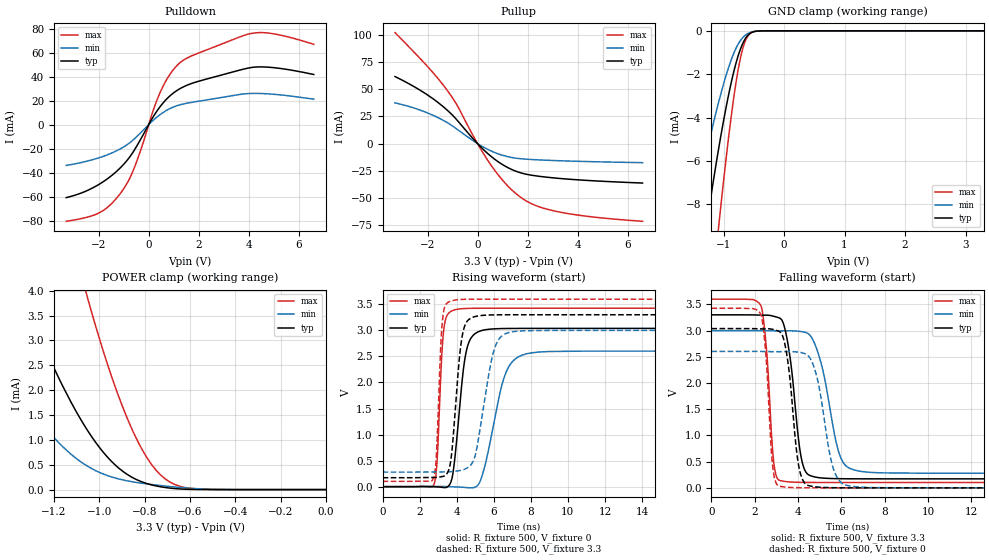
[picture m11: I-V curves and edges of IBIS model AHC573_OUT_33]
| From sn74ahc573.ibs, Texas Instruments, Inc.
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[Model]   AHC573_OUT_33
Model_type  3-state
Enable   Active-Low
Vref =   0.0
Rref =   1000
Cref =   50p
Vmeas =   1.65
| variable   typ   min   max
C_comp   2.19pF   1.91pF   2.36pF
| C_pullup   3.29pF   2.02pF   4.04pF
| C_pulldown   2.75pF   1.99pF   3.57pF
| C_tri-state   2.19pF   1.91pF   2.36pF
[Temperature Range]   40   100   -40
| Ambient temperature   25   85   -40
[Voltage range]   3.3   3   3.6
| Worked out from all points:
|   slope of the pulldown table from 0 to 0.495 V, typ, clamps not added: 30.9 ohm
|   slope of the pullup table from 0 to 0.495 V, typ, clamps not added: 45.5 ohm
|   GND clamp passes 1 mA (typ) near -0.74 V on its own axis
|   POWER clamp passes 1 mA (typ) near -1.02 V on its own axis
|   rising waveform, R_fixture 500, V_fixture 0: 20-80 % time 514ps typ, 946ps min, 263ps max; typ from 0 V to 3.04 V
|   falling waveform, R_fixture 500, V_fixture 3.3: 20-80 % time 499ps typ, 776ps min, 325ps max; typ from 3.3 V to 0.172 V
|   rising waveform, R_fixture 500, V_fixture 3.3: 20-80 % time 436ps typ, 764ps min, 239ps max; typ from 0.172 V to 3.3 V
|   falling waveform, R_fixture 500, V_fixture 0: 20-80 % time 439ps typ, 642ps min, 297ps max; typ from 3.04 V to 0 V
[GND Clamp]
| AHC573_OUT_33
|   Voltage   I(typ)   I(min)   I(max)
-3.3V     -60.86mA   -39.73mA   -82.26mA
-1.52V    -13.86mA   -8.821mA   -21.9mA
-1.28V    -8.984mA   -5.626mA   -14.64mA
-1.1V     -5.753mA   -3.504mA   -9.558mA
-1.07V    -5.258mA   -3.179mA   -8.754mA
-905mV    -2.803mA   -1.596mA   -4.662mA
-835mV    -1.937mA   -1.066mA   -3.167mA
-780mV    -1.355mA   -728.6uA   -2.148mA
-690mV    -630uA     -338.2uA   -897.4uA
-590mV    -183.7uA   -113uA     -211.6uA
-375mV    -3.862uA   -2.975uA   -1.96uA
3.3V      10.72nA    15.77nA    51.49nA
[POWER Clamp]
| AHC573_OUT_33
|   Voltage   I(typ)   I(min)   I(max)
-3.3V     44.46mA    27.37mA    76.31mA
-1.605V   7.526mA    3.914mA    16.22mA
-1.335V   3.908mA    1.826mA    9.462mA
-1.18V    2.261mA    949.9uA    6.178mA
-1.065V   1.287mA    509.3uA    4.083mA
-1.05V    1.179mA    466.7uA    3.834mA
-960mV    635.2uA    276.2uA    2.471mA
-865mV    272.4uA    166.5uA    1.311mA
-790mV    121.4uA    114.1uA    643.8uA
-710mV    42.77uA    72.33uA    217.8uA
-575mV    2.489uA    19.9uA     14.31uA
-48.03fV  10.72nA    1.614nA    79.93nA
[Pulldown]
| AHC573_OUT_33
|   Voltage   I(typ)   I(min)   I(max)
-3.3V     -60.82mA   -34mA      -80.56mA
-1.955V   -49.36mA   -27.41mA   -73.22mA
-1.53V    -43.23mA   -24.12mA   -66.71mA
-1.095V   -35.12mA   -19.74mA   -56.23mA
-580mV    -21.4mA    -11.96mA   -36.16mA
195mV     7.045mA    3.905mA    12.83mA
505mV     16.27mA    9.059mA    28.99mA
905mV     24.95mA    13.91mA    43.54mA
1.345V    31mA       17.03mA    53.09mA
4.23V     47.88mA    26mA       76.33mA
5.125V    47.14mA    25.02mA    75.15mA
6.6V      41.74mA    21.26mA    66.86mA
[Pullup]
| AHC573_OUT_33
|   Voltage   I(typ)   I(min)   I(max)
-3.3V     61.59mA    37.44mA    102mA
-2.18V    47.37mA    29.8mA     75.34mA
-1.31V    32.68mA    20.57mA    51.94mA
-830mV    21.86mA    13.38mA    35.7mA
-40mV     989.5uA    591.7uA    1.624mA
495mV     -10.88mA   -6.291mA   -18.35mA
1.08V     -20.42mA   -11.28mA   -35.71mA
1.66V     -26.4mA    -13.78mA   -48.23mA
2.305V    -29.58mA   -14.83mA   -56.72mA
3.225V    -31.92mA   -15.73mA   -62.67mA
4.61V     -34.17mA   -16.65mA   -67.45mA
6.6V      -36.27mA   -17.55mA   -71.43mA
[Ramp]
| AHC573_OUT_33
| variable   typ   min   max
dV/dt_r   1.83/5.21E-10   1.58/9.54E-10   2.06/2.67E-10
dV/dt_f   1.88/5.01E-10   1.63/7.78E-10   2.10/3.30E-10
R_load = 500
[Rising Waveform]
| AHC573_OUT_33
R_fixture =   500
C_fixture =   0
L_fixture =   0
V_fixture =   0
V_fixture_min = 0
V_fixture_max = 0
|   Time   V(typ)   V(min)   V(max)
0s        717.3pV    1.212nV    402.8pV
2.775ns   -836.6uV   4.547mV    44.17mV
2.94ns    -4.688mV   4.776mV    497mV
3.315ns   -17.22mV   3.17mV     3.053V
4ns       903mV      -5.604mV   3.404V
4.405ns   2.371V     -14.01mV   3.419V
4.785ns   2.861V     -22.99mV   3.423V
6.695ns   3.036V     2.223V     3.425V
8.005ns   3.038V     2.567V     3.425V
50ns      3.038V     2.603V     3.425V
[Falling Waveform]
| AHC573_OUT_33
R_fixture =   500
C_fixture =   0
L_fixture =   0
V_fixture =   3.3
V_fixture_min = 3
V_fixture_max = 3.6
|   Time   V(typ)   V(min)   V(max)
0s        3.3V       3V         3.6V
2.305ns   3.294V     3V         3.456V
2.875ns   3.273V     2.995V     491.4mV
3.21ns    3.22V      2.995V     134mV
3.605ns   2.558V     2.996V     113.2mV
4.185ns   498.8mV    2.979V     105mV
4.905ns   198mV      2.595V     102.7mV
5.94ns    174.7mV    605.7mV    102.1mV
7.005ns   172.1mV    307.7mV    102mV
50ns      171.7mV    279.8mV    102mV
[Rising Waveform]
| AHC573_OUT_33
R_fixture =   500
C_fixture =   0
L_fixture =   0
V_fixture =   3.3
V_fixture_min = 3
V_fixture_max = 3.6
|   Time   V(typ)   V(min)   V(max)
0s        171.7mV    279.8mV    102mV
2.74ns    175.5mV    282.5mV    161.1mV
2.895ns   177.9mV    282.7mV    557.7mV
3.25ns    196.4mV    283.2mV    3.255V
3.86ns    1.185V     293.4mV    3.579V
4.5ns     3.142V     346.6mV    3.597V
5.025ns   3.268V     640mV      3.599V
6.045ns   3.298V     2.656V     3.6V
7.005ns   3.3V       2.974V     3.6V
50ns      3.3V       3V         3.6V
[Falling Waveform]
| AHC573_OUT_33
R_fixture =   500
C_fixture =   0
L_fixture =   0
V_fixture =   0
V_fixture_min = 0
V_fixture_max = 0
|   Time   V(typ)   V(min)   V(max)
0s        3.038V     2.603V     3.425V
2.305ns   3.032V     2.602V     3.282V
2.83ns    3.023V     2.598V     403.5mV
3.205ns   2.958V     2.598V     25.88mV
3.545ns   2.358V     2.6V       10.39mV
4.065ns   345.7mV    2.586V     3.171mV
4.72ns    24.19mV    2.324V     869.2uV
5.63ns    3.096mV    365.8mV    158.7uV
6.56ns    539.4uV    25.47mV    29.28uV
50ns      1.856nV    10.26nV    588.2pV
